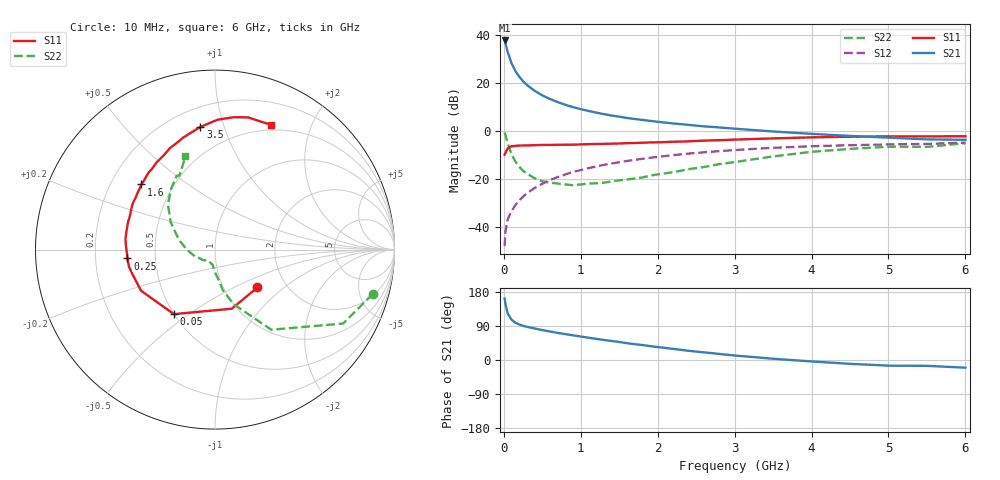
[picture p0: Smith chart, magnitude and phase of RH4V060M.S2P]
! SIEMENS Small Signal Semiconductors
! BFR106
! Si NPN RF Bipolar Junction Transistor in SOT23
! VCE = 4 V  IC = 60 mA
! Common Emitter S-Parameters:  August  1996
# GHz  S  MA  R  50
!  f  S11  S21  S12  S22
! GHz  MAG  ANG  MAG  ANG  MAG  ANG  MAG  ANG
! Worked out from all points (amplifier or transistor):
!   36 points, 10 MHz to 6 GHz, reference 50 ohm
!   highest |S21| = 37.6 dB at 10 MHz (marker M1)
!   |S21| within 3 dB of that: start of sweep to 35.84 MHz
!   unconditionally stable (mu >= 1): 227.9 MHz to 2.382 GHz
!   at 250 MHz: K = 1.02, MAG = 23.2 dB, |S12| = -27.5 dB
!   at 1.4 GHz: K = 1.06, MAG = 8.5 dB, |S12| = -13.7 dB
!   at 6 GHz: K = 0.99, MSG = 0.6 dB, |S12| = -5.0 dB
!   S11 on the Smith chart (normalised r, x): 10 MHz: 1.43, -0.67; 50 MHz: 0.50, -0.44; 250 MHz: 0.34, -0.04; 1.6 GHz: 0.33, +0.34; 3.5 GHz: 0.32, +0.84; 6 GHz: 0.44, +1.45
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0.01  0.3166 -41.8  75.77 162.4  0.0039 83.5  0.9132 -15.7
0.02  0.3424 -74.1  67.27 148.6  0.0076 71.3  0.8241 -30.0
0.05  0.4263 -122.5  43.81 123.1  0.0142 61.3  0.5456 -54.9
0.1  0.4712 -150.9  25.38 106.4  0.021 63.3  0.3207 -71.2
0.15  0.4794 -162.9  17.45 98.3  0.028 66.2  0.2274 -79.4
0.2  0.4887 -168.9  13.3 93.8  0.035 68.7  0.1773 -82.2
0.25  0.4901 -174.2  10.68 90.1  0.042 70.5  0.1444 -86.6
0.3  0.4907 -177.3  8.939 87.6  0.0493 71.7  0.1274 -89.8
0.4  0.4971 177.2  6.773 83.2  0.0637 72.5  0.1017 -94.5
0.5  0.5024 173.2  5.432 79.0  0.0781 72.4  0.0878 -98.1
0.6  0.5036 168.9  4.556 75.2  0.0932 71.9  0.0819 -101.9
0.7  0.5056 165.1  3.932 71.5  0.1076 71.0  0.0792 -107.3
0.9  0.5095 158.7  3.09 65.1  0.1374 68.6  0.0728 -115.5
1.1  0.5221 152.4  2.574 58.8  0.165 66.0  0.0791 -124.9
1.3  0.5286 146.6  2.206 52.9  0.1929 63.0  0.0821 -133.9
1.6  0.5474 138.5  1.836 44.4  0.233 58.6  0.096 -147.6
2.2  0.5854 123.6  1.41 29.4  0.3081 49.4  0.1356 -171.8
2.8  0.6308 109.8  1.164 16.0  0.3734 40.0  0.1997 166.6
3.5  0.6884 96.8  0.96 3.3  0.4384 29.4  0.2897 148.3
4.5  0.7445 82.1  0.775 -10.1  0.496 14.8  0.4157 126.3
5.5  0.7574 70.1  0.657 -15.4  0.5278 5.4  0.458 115.5
6  0.7625 65.9  0.644 -20.3  0.5611 -1.6  0.5455 107.6
